PROGRAM MAIN
VAR
	bSimulation					: BOOL:=TRUE; (* Enables/disables simulation of data update/change *)
	tSimulation					: TIME:=T#2S; (* Cycle time of simulated data update/change *)
	fbTimer						: TON;
	tT							: T_UtcTime;
	
	bReplaceBufferedMX			: BOOL; (* Toggles bReplaceBufferedMX property of urcb201 *)
	bOverwriteSameCycleChanges	: BOOL; (* Toggles bOverwriteSameCycleChanges property of urcb301 *)
END_VAR

P_IEC61850MAIN();

fbIED.IEDLD1.LLN0.urcb201.Server.bReplaceBufferedMX:= bReplaceBufferedMX;
fbIED.IEDLD1.LLN0.urcb301.Server.bOverwriteSameCycleChanges:= bOverwriteSameCycleChanges;

fbTimer(IN:=bSimulation, PT:=tSimulation);
IF fbTimer.Q THEN(* Simulate server data update *)
	fbTimer(IN:=FALSE);
	fbTimer(IN:=bSimulation);

	fbIEDServer.GetSystemTime(ipAA:=0, tT=>tT);
	
	(* Simulate "IEDLD1/LLN0.DS1" member value change *)
	fbIED.IEDLD1.LEDGGIO1.SPCSO1.t.tValue:= tT;
	fbIED.IEDLD1.LEDGGIO1.SPCSO1.stVal.bValue:= NOT fbIED.IEDLD1.LEDGGIO1.SPCSO1.stVal.bValue;
	fbIED.IEDLD1.LEDGGIO2.SPCSO1.t.tValue:= tT;
	fbIED.IEDLD1.LEDGGIO2.SPCSO1.stVal.bValue:= NOT fbIED.IEDLD1.LEDGGIO2.SPCSO1.stVal.bValue;
	fbIED.IEDLD1.LEDGGIO3.SPCSO1.t.tValue:= tT;
	fbIED.IEDLD1.LEDGGIO3.SPCSO1.stVal.bValue:= NOT fbIED.IEDLD1.LEDGGIO3.SPCSO1.stVal.bValue;
	fbIED.IEDLD1.LEDGGIO4.SPCSO1.t.tValue:= tT;
	fbIED.IEDLD1.LEDGGIO4.SPCSO1.stVal.bValue:= NOT fbIED.IEDLD1.LEDGGIO4.SPCSO1.stVal.bValue;
	fbIED.IEDLD1.LEDGGIO5.SPCSO1.t.tValue:= tT;
	fbIED.IEDLD1.LEDGGIO5.SPCSO1.stVal.bValue:= NOT fbIED.IEDLD1.LEDGGIO5.SPCSO1.stVal.bValue;
	fbIED.IEDLD1.LEDGGIO6.SPCSO1.t.tValue:= tT;
	fbIED.IEDLD1.LEDGGIO6.SPCSO1.stVal.bValue:= NOT fbIED.IEDLD1.LEDGGIO6.SPCSO1.stVal.bValue;
	fbIED.IEDLD1.LEDGGIO7.SPCSO1.t.tValue:= tT;
	fbIED.IEDLD1.LEDGGIO7.SPCSO1.stVal.bValue:= NOT fbIED.IEDLD1.LEDGGIO7.SPCSO1.stVal.bValue;
	fbIED.IEDLD1.LEDGGIO8.SPCSO1.t.tValue:= tT;
	fbIED.IEDLD1.LEDGGIO8.SPCSO1.stVal.bValue:= NOT fbIED.IEDLD1.LEDGGIO8.SPCSO1.stVal.bValue;

	(* Simulate "IEDLD1/LLN0.DS2" member value change *)
	fbIED.IEDLD1.MMXU1.TotW.t.tValue:= tT;
	fbIED.IEDLD1.MMXU1.TotW.mag.f.fValue:= fbIED.IEDLD1.MMXU1.TotW.mag.f.fValue + 0.1;
	
	(* Simulate "IEDLD1/LLN0.DS3" member value change *)
	fbIED.IEDLD1.XCBR1.Pos.t.tValue:= tT;
	IF fbIED.IEDLD1.XCBR1.Pos.stVal.eValue = E_AcsiDbpos.On THEN
		fbIED.IEDLD1.XCBR1.Pos.stVal.eValue:= E_AcsiDbpos.Off;
	ELSE
		fbIED.IEDLD1.XCBR1.Pos.stVal.eValue:= E_AcsiDbpos.On;
	END_IF
	fbIED.IEDLD1.XCBR1.Pos.q.OldData:= NOT fbIED.IEDLD1.XCBR1.Pos.q.OldData;
	fbIED.IEDLD1.XCBR1.Pos.q.eValidity:= SEL(fbIED.IEDLD1.XCBR1.Pos.q.OldData, E_AcsiQualityValidity.Good, E_AcsiQualityValidity.Questionable);
END_IF

END_PROGRAM
